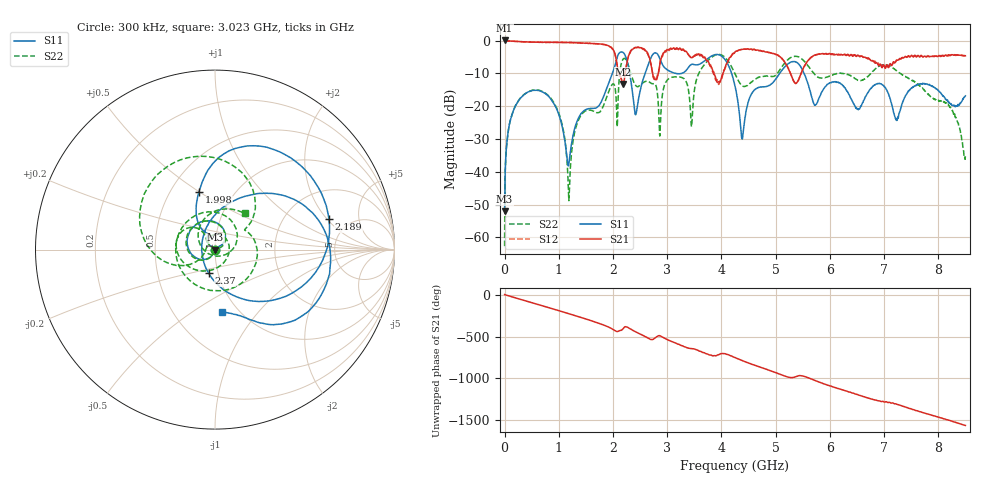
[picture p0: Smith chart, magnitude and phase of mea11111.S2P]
!Agilent Technologies,E5071B,MY42402595,A.08.01
!Date: Tue Jan 02 09:36:45 2001
!Data & Calibration Information:
!Freq	S11:SOLT2(ON)	S21:SOLT2(ON)	S12:SOLT2(ON)	S22:SOLT2(ON)
# Hz S dB R 50
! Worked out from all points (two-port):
!   1601 points, 300 kHz to 8.5 GHz, reference 50 ohm
!   highest |S21| = 0.04 dB at 300 kHz (marker M1); lowest = -13.2 dB at 2.184 GHz (marker M2)
!   |S21| within 3 dB of the highest: start of sweep to 2.009 GHz; 4.313 GHz to 4.679 GHz (366.4 MHz wide, 8.15 % of centre)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
!   lowest |S11| = -52.0 dB at 300 kHz (marker M3), VSWR 1.01, Z = 50.2 - j0.0373 ohm
!   |S11| at or under -10 dB: start of sweep to 1.988 GHz; 4.187 GHz to 5.076 GHz (888.5 MHz wide, 19.2 % of centre); 5.525 GHz to end of sweep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
!   |S22| runs from -62.7 to -4.2 dB; largest |S21 - S12| = 0.049
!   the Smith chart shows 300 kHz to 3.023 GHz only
!   S11 on the Smith chart (normalised r, x): 300 kHz: 1.00, -0.00; 1.998 GHz: 0.69, +0.50; 2.189 GHz: 3.52, +2.09; 2.37 GHz: 0.90, -0.24; 3.023 GHz: 0.85, -0.67
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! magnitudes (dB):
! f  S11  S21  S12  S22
! 300 kHz  -52.0  0.0  0.0  -62.7
! 74.67 MHz  -26.8  -0.1  -0.1  -26.8
! 297.8 MHz  -17.4  -0.3  -0.3  -17.4
! 898.1 MHz  -18.9  -0.5  -0.6  -18.6
! 1.185 GHz  -37.7  -0.6  -0.6  -48.8
! 1.419 GHz  -22.1  -0.8  -0.8  -22.6
! 1.998 GHz  -9.6  -2.7  -2.8  -13.2
! 2.184 GHz  -3.6  -13.2  -13.4  -5.7
! 2.189 GHz  -3.6  -13.2  -13.2  -5.6
! 2.37 GHz  -17.3  -2.6  -2.4  -12.1
! 2.837 GHz  -4.5  -9.8  -9.8  -19.9
! 3.023 GHz  -9.2  -2.8  -2.8  -11.7
! 3.448 GHz  -7.3  -5.2  -5.4  -26.3
! 3.799 GHz  -4.9  -7.9  -7.4  -5.3
! 4.25 GHz  -13.8  -3.5  -3.5  -10.1
! 4.388 GHz  -29.8  -2.7  -2.7  -13.9
! 4.58 GHz  -15.6  -2.8  -2.7  -12.3
! 5.27 GHz  -6.6  -9.9  -9.9  -5.3
! 5.669 GHz  -17.4  -4.9  -5.0  -9.3
! 7.087 GHz  -16.5  -8.2  -7.7  -7.6
! 8.192 GHz  -19.0  -4.3  -4.7  -19.7
! 8.5 GHz  -16.9  -4.6  -4.6  -35.3
